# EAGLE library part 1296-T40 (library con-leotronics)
1.27mm SINGLE ROW FEMALE SOCKET Source: http://www.leotronics.co.uk/Conexcon/Data%20Sheets/sec.%20A/1296ing.pdf
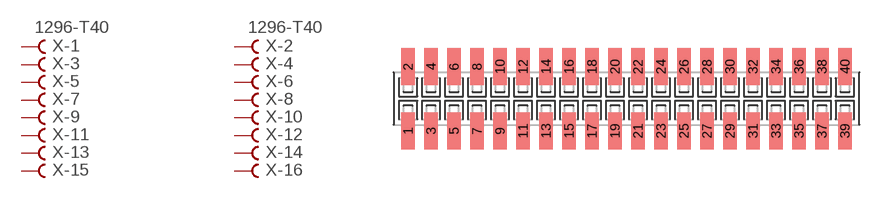
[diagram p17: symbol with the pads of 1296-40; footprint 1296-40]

Designator prefix X; gates -1=FVAL -2=FVAL -3=F -4=F -5=F -6=F -7=F -8=F -9=F -10=F -11=F -12=F -13=F -14=F -15=F -16=F -17=F -18=F -19=F -20=F -21=F -22=F -23=F -24=F -25=F -26=F -27=F -28=F -29=F -30=F -31=F -32=F -33=F -34=F -35=F -36=F -37=F -38=F -39=F -40=F

## 1296-T40 (OC_FARNELL: unknown; OC_NEWARK: unknown)  [1296-40]
1  -1:B  pas
2  -2:B  pas
3  -3:B  pas
4  -4:B  pas
5  -5:B  pas
6  -6:B  pas
7  -7:B  pas
8  -8:B  pas
9  -9:B  pas
10  -10:B  pas
11  -11:B  pas
12  -12:B  pas
13  -13:B  pas
14  -14:B  pas
15  -15:B  pas
16  -16:B  pas
17  -17:B  pas
18  -18:B  pas
19  -19:B  pas
20  -20:B  pas
21  -21:B  pas
22  -22:B  pas
23  -23:B  pas
24  -24:B  pas
25  -25:B  pas
26  -26:B  pas
27  -27:B  pas
28  -28:B  pas
29  -29:B  pas
30  -30:B  pas
31  -31:B  pas
32  -32:B  pas
33  -33:B  pas
34  -34:B  pas
35  -35:B  pas
36  -36:B  pas
37  -37:B  pas
38  -38:B  pas
39  -39:B  pas
40  -40:B  pas

## Footprint 1296-40 (pad centres in mm)
1.27mm SINGLE ROW FEMALE SOCKET Source: http://www.leotronics.co.uk/Conexcon/Data%20Sheets/sec.%20A/1296ing.pdf
smd 0.76 x 2.05: 1 -12.065,-1.78; 2 -12.065,1.78; 3 -10.795,-1.78; 4 -10.795,1.78; 5 -9.525,-1.78; 6 -9.525,1.78; 7 -8.255,-1.78; 8 -8.255,1.78; 9 -6.985,-1.78; 10 -6.985,1.78; 11 -5.715,-1.78; 12 -5.715,1.78; 13 -4.445,-1.78; 14 -4.445,1.78; 15 -3.175,-1.78; 16 -3.175,1.78; 17 -1.905,-1.78; 18 -1.905,1.78; 19 -0.635,-1.78; 20 -0.635,1.78; 21 0.635,-1.78; 22 0.635,1.78; 23 1.905,-1.78; 24 1.905,1.78; 25 3.175,-1.78; 26 3.175,1.78; 27 4.445,-1.78; 28 4.445,1.78; 29 5.715,-1.78; 30 5.715,1.78; 31 6.985,-1.78; 32 6.985,1.78; 33 8.255,-1.78; 34 8.255,1.78; 35 9.525,-1.78; 36 9.525,1.78; 37 10.795,-1.78; 38 10.795,1.78; 39 12.065,-1.78; 40 12.065,1.78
